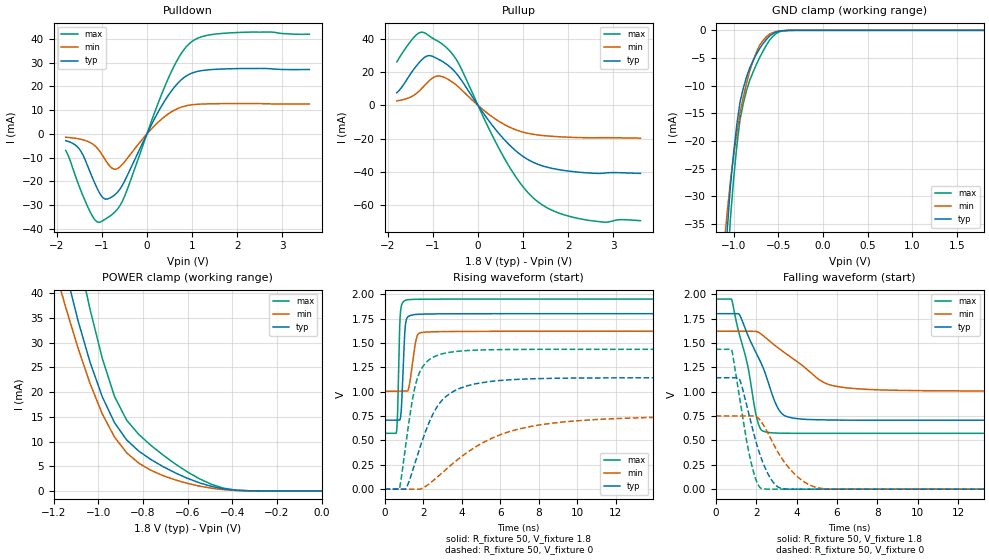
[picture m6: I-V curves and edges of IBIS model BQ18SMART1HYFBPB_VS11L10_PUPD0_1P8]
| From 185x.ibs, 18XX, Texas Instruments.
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|   Model Cell BQ18SMART1HYFBPB_VS11L10_PUPD0_1P8
|BQ18SMART1HYFBPB_VS11L10_PUPD0_1P8
[Model]   BQ18SMART1HYFBPB_VS11L10_PUPD0_1P8
Model_type   I/O
Polarity   Non-Inverting
Enable   Active-Low
Vinl =  0.63
Vinh =  1.17
Cref =  15pF
Rref =  100.0000M
Vref =  0V
Vmeas =  0.9
C_comp   0.9029199p   0.7983694p   1.014934p
[Model Spec]
Vinl   0.63   0.567   0.6825
Vinh   1.17   1.053   1.2675
[Temperature Range]   25   125   -40
[Voltage Range]   1.8   1.62   1.95
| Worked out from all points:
|   slope of the pulldown table from 0 to 0.27 V, typ, clamps not added: 27.2 ohm
|   slope of the pullup table from 0 to 0.27 V, typ, clamps not added: 26 ohm
|   GND clamp passes 1 mA (typ) near -0.59 V on its own axis
|   POWER clamp passes 1 mA (typ) near -0.50 V on its own axis
|   rising waveform, R_fixture 50, V_fixture 1.8: 20-80 % time 143ps typ, 261ps min, 100ps max; typ from 0.708 V to 1.8 V
|   rising waveform, R_fixture 50, V_fixture 0: 20-80 % time 1.48ns typ, 3.7ns min, 734ps max; typ from 0 V to 1.14 V
|   falling waveform, R_fixture 50, V_fixture 1.8: 20-80 % time 1.29ns typ, 2.29ns min, 851ps max; typ from 1.8 V to 0.708 V
|   falling waveform, R_fixture 50, V_fixture 0: 20-80 % time 953ps typ, 1.41ns min, 720ps max; typ from 1.14 V to 0 V
| Nom Voltages:
|   BIASFET=1.8, VBBNW=1.1, VDD=1.1, VDDS=1.8, VSS=0, VSSS=0
| Min Voltages:
|   BIASFET=1.62, VBBNW=0.99, VDD=0.99, VDDS=1.62, VSS=0, VSSS=0
| Max Voltages:
|   BIASFET=1.95, VBBNW=1.21, VDD=1.21, VDDS=1.95, VSS=0, VSSS=0
[POWER_clamp]
|   voltage   I(typ)   I(min)   I(max)
-1.8V     196.8mA    157.5mA    250.4mA
-1.164V   48mA       40.06mA    64.23mA
-1.127V   41.11mA    34.43mA    55.95mA
-1.109V   37.83mA    31.72mA    51.94mA
-1.055V   28.88mA    24.15mA    40.47mA
-981.8mV  19.06mA    15.6mA     26.85mA
-927.3mV  13.83mA    10.93mA    19.15mA
-872.7mV  10.34mA    7.72mA     14.33mA
-763.6mV  6.344mA    4.165mA    9.211mA
-600mV    2.546mA    1.527mA    3.832mA
-436.4mV  402.5uA    253uA      527.5uA
0V        291.8pA    1.073nA    4.224nA
[Pulldown]
|   voltage   I(typ)   I(min)   I(max)
-1.8V     -2.835mA   -1.376mA   -6.938mA
-1.473V   -6.994mA   -2.229mA   -23.44mA
-1.2V     -18.79mA   -4.282mA   -34.89mA
-1.036V   -25.33mA   -7.531mA   -37.14mA
-872.7mV  -27.39mA   -12.36mA   -35.28mA
-654.5mV  -24.59mA   -14.63mA   -31.68mA
-490.9mV  -19.69mA   -11.65mA   -26.08mA
381.8mV   13.54mA    7.117mA    19.32mA
654.5mV   20.72mA    10.44mA    30.48mA
927.3mV   25mA       12.07mA    37.79mA
1.636V    27.3mA     12.74mA    42.26mA
3.6V      27.12mA    12.64mA    41.97mA
[Pullup]
|   voltage   I(typ)   I(min)   I(max)
-1.8V     7.614mA    2.74mA     26.22mA
-1.527V   17.69mA    4.626mA    37.43mA
-1.309V   25.69mA    8.541mA    43.72mA
-1.036V   29.87mA    15.94mA    41.05mA
-818.2mV  26.95mA    17.52mA    37.49mA
-490.9mV  19.61mA    12.45mA    28.08mA
545.5mV   -19.54mA   -10.94mA   -30.03mA
927.3mV   -29.38mA   -15.56mA   -46.58mA
1.255V    -34.7mA    -17.56mA   -56.51mA
1.691V    -38.25mA   -18.74mA   -63.85mA
2.291V    -40.42mA   -19.45mA   -68.55mA
3.6V      -41.01mA   -19.75mA   -69.5mA
[GND_clamp]
|   voltage   I(typ)   I(min)   I(max)
-1.8V     -274mA     -200.4mA   -365.5mA
-1.109V   -45.37mA   -39.32mA   -55.85mA
-1.073V   -36.45mA   -33.1mA    -44.39mA
-1.036V   -28.3mA    -27.35mA   -34.22mA
-1V       -22.14mA   -22.69mA   -26.92mA
-927.3mV  -12.91mA   -14.91mA   -16.03mA
-854.5mV  -8.387mA   -9.532mA   -10.83mA
-781.8mV  -5.484mA   -5.512mA   -7.535mA
-709.1mV  -3.298mA   -2.71mA    -4.931mA
-600mV    -1.058mA   -705.2uA   -1.831mA
-381.8mV  -13.32uA   -12.31uA   -19.39uA
1.8V      291.8pA    820.3nA    4.087nA
[Ramp]
| variable   typ   min   max
dV/dt_f 0.65735248/1.2928228n  0.3698284/2.2967163n 0.82887642/0.8537792n
dV/dt_r 0.69452928/1.4830192n 0.45781578/3.7933581n 0.86939267/0.73665477n
R_load = 50
[Rising Waveform]
R_fixture = 50
V_fixture = 1.8
V_fixture_min = 1.62
V_fixture_max = 1.95
|   time   V(typ)   V(min)   V(max)
0s        708mV      1.005V     573mV
615.6ps   708mV      1.005V     588.6mV
673.8ps   708mV      1.005V     782.8mV
765.9ps   708mV      1.005V     1.561V
812.6ps   723.4mV    1.005V     1.792V
1.085ns   1.694V     1.005V     1.937V
1.271ns   1.776V     1.053V     1.944V
1.652ns   1.793V     1.549V     1.947V
1.918ns   1.795V     1.607V     1.948V
17.87ns   1.8V       1.62V      1.95V
[Rising Waveform]
R_fixture = 50
V_fixture = 0
V_fixture_min = 0
V_fixture_max = 0
|   time   V(typ)   V(min)   V(max)
0s        0V         0V         0V
763.6ps   0V         0V         0V
1.096ns   0V         0V         454.6mV
1.411ns   162.7mV    0V         877.4mV
1.642ns   307.9mV    0V         1.099V
2.011ns   530.2mV    15.36mV    1.265V
2.684ns   832.8mV    115.1mV    1.368V
4.193ns   1.054V     363.5mV    1.421V
7.393ns   1.13V      635.8mV    1.434V
18.03ns   1.143V     745.1mV    1.434V
[Falling Waveform]
R_fixture = 50
V_fixture = 1.8
V_fixture_min = 1.62
V_fixture_max = 1.95
|   time   V(typ)   V(min)   V(max)
0s        1.8V       1.62V      1.95V
797.8ps   1.8V       1.62V      1.941V
1.186ns   1.786V     1.62V      1.575V
1.583ns   1.582V     1.62V      1.267V
2.026ns   1.388V     1.616V     733.9mV
2.356ns   1.241V     1.574V     594.4mV
3.121ns   816.1mV    1.444V     574.5mV
3.857ns   728.3mV    1.335V     572.9mV
6.485ns   708mV      1.039V     572.6mV
17.87ns   707.6mV    1.006V     572.6mV
[Falling Waveform]
R_fixture = 50
V_fixture = 0
V_fixture_min = 0
V_fixture_max = 0
|   time   V(typ)   V(min)   V(max)
0s        1.143V     751.6mV    1.435V
793.2ps   1.143V     751.6mV    1.426V
1.188ns   1.121V     751.6mV    928.9mV
1.657ns   756.3mV    751.6mV    361.3mV
1.98ns    496mV      747.3mV    104.5mV
2.253ns   317.4mV    692.5mV    7.133mV
3.099ns   20.55mV    372.2mV    0V
4.016ns   0V         133.3mV    0V
5.093ns   0V         12.26mV    0V
18.03ns   0V         0V         0V
